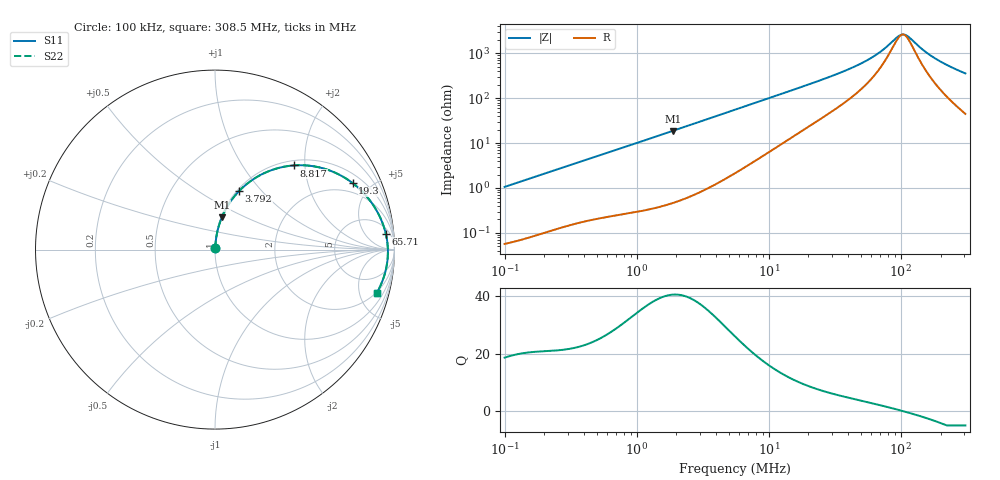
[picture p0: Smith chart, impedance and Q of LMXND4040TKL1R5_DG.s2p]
! LMXND4040TKL1R5_DG  S-PARAMETER MODEL  ( General Type )
! Model Generated by TAIYO YUDEN Corporation (https://www.yuden.co.jp/en/)
! Version 1.0
! TAIYO YUDEN Control No. 191023NI43SB-FBB
! Copyright(c) 2019 TAIYO YUDEN CO.,LTD. All Rights Reserved.
! Product Description (link to TY-COMPAS)
! https://ds.yuden.co.jp/TYCOMPAS/or/detail?pn=LMXND4040TKL1R5NDG&u=M
! Products Name : Inductors
! Characteristics :
!  Inductance : 1.5 uH , SRF(min) : 75 MHz , DC Resistance(max) : 0.0444 Ohm
!  Rated Current : Saturation :3300 mA , Temp Rise : 2400 mA (40 degC)
!  Case Size : 4.0 x 4.0 / 0.157 x 0.157 [mm/inch] , Thickness : 1.8 / 0.071 [mm/inch]
!  (Conditions: Temperature = 25 degC , DC Bias Current/Voltage = 0A / 0V)
! External Node Assignments :
!  1  o---GGG---o  2
! GND o---------o GND
! Frequency Range : 0.1MHz  -  308.54851MHz  [ 402 STEP ]
# MHz S RI R 50
! Freq[MHz].  S11 Real  S11 Imag  S21 Real  S21 Imag  S12 Real  S12 Imag  S22 Real  S22 Imag
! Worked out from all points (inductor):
!   401 points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, 100 kHz to 308.5 MHz, reference 50 ohm
!   read as one part in series: L = 1.68 uH near 104.1 kHz
!   highest Q = 40.5 at 1.878 MHz (marker M1), where L = 1.59 uH
!   self-resonance near 103.6 MHz
!   S11 on the Smith chart (normalised r, x): 100 kHz: 1.00, +0.02; 3.792 MHz: 1.02, +0.76; 8.817 MHz: 1.10, +1.76; 19.3 MHz: 1.43, +3.87; 65.71 MHz: 8, +17; 308.5 MHz: 1.89, -7.06
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0.1  0.000681 0.0106  0.9993 -0.0106  0.9993 -0.0106  0.000681 0.0106
0.384115  0.00327 0.0391  0.9967 -0.0391  0.9967 -0.0391  0.00327 0.0391
0.807652  0.00914 0.0803  0.9909 -0.0803  0.9909 -0.0803  0.00914 0.0803
1.475446  0.0248 0.1433  0.9752 -0.1433  0.9752 -0.1433  0.0248 0.1433
1.8776  0.0381 0.1795  0.9619 -0.1795  0.9619 -0.1795  0.0381 0.1795
3.792441  0.1325 0.3244  0.8675 -0.3244  0.8675 -0.3244  0.1325 0.3244
5.667415  0.2505 0.4142  0.7495 -0.4142  0.7495 -0.4142  0.2505 0.4142
8.816533  0.4398 0.469  0.5602 -0.469  0.5602 -0.469  0.4398 0.469
12.65661  0.6077 0.4512  0.3923 -0.4512  0.3923 -0.4512  0.6077 0.4512
19.29776  0.7668 0.3706  0.2332 -0.3706  0.2332 -0.3706  0.7668 0.3706
21.33651  0.796 0.3466  0.204 -0.3466  0.204 -0.3466  0.796 0.3466
41.39926  0.9166 0.1869  0.0834 -0.1869  0.0834 -0.1869  0.9166 0.1869
53.75212  0.9398 0.1301  0.0602 -0.1301  0.0602 -0.1301  0.9398 0.1301
65.70958  0.9516 0.089  0.0484 -0.089  0.0484 -0.089  0.9516 0.089
81.95682  0.9596 0.0454  0.0404 -0.0454  0.0404 -0.0454  0.9596 0.0454
98.19624  0.9629 0.0104  0.0371 -0.0104  0.0371 -0.0104  0.9629 0.0104
108.5704  0.9634 -0.00912  0.0366 0.00912  0.0366 0.00912  0.9634 -0.00912
117.6534  0.9632 -0.0248  0.0368 0.0248  0.0368 0.0248  0.9632 -0.0248
149.7216  0.9592 -0.0733  0.0408 0.0733  0.0408 0.0733  0.9592 -0.0733
179.3883  0.9521 -0.1116  0.0479 0.1116  0.0479 0.1116  0.9521 -0.1116
232.9148  0.9342 -0.1715  0.0658 0.1715  0.0658 0.1715  0.9342 -0.1715
308.5485  0.9006 -0.2425  0.0994 0.2425  0.0994 0.2425  0.9006 -0.2425
